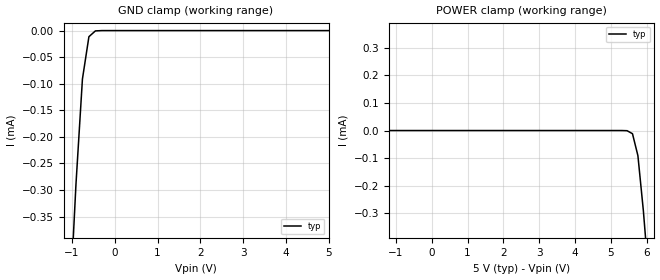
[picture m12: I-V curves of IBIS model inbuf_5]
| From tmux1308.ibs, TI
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| inbuf_5
[Model]   inbuf_5
Model_type   Input
Vinl = 0.95
Vinh = 1.25
|   typ   min   max
C_comp   4.014581e-14   NA   NA
[Voltage Range]   5   NA   NA
[Temperature Range]   27   NA   NA
[Power Clamp Reference]   5   NA   NA
[GND Clamp Reference]   0   NA   NA
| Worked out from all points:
|   GND clamp passes 1 mA (typ) near -1.33 V on its own axis
|   POWER clamp passes 1 mA (typ) near -3.64 V on its own axis
[GND Clamp]
|   Voltage   I(typ)   I(min)   I(max)
-10V      -57.25mA   NA         NA
-1.061V   -532.2uA   NA         NA
-909.1mV  -289.4uA   NA         NA
-757.6mV  -91.09uA   NA         NA
-606.1mV  -11.52uA   NA         NA
-454.5mV  -609.8nA   NA         NA
5V        72.6pA     NA         NA
[POWER Clamp]
|   Voltage   I(typ)   I(min)   I(max)
-5V       203.6mA    NA         NA
-3.636V   871.3uA    NA         NA
-3.485V   26.43uA    NA         NA
-3.333V   20.69uA    NA         NA
-2.727V   9.699uA    NA         NA
-1.97V    68.26nA    NA         NA
5.455V    -609.8nA   NA         NA
5.606V    -11.52uA   NA         NA
5.758V    -91.09uA   NA         NA
5.909V    -289.4uA   NA         NA
6.061V    -532.2uA   NA         NA
10V       -7.717mA   NA         NA
